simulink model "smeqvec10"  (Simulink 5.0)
settings: Solver=ode45  StartTime=0.0  StopTime=5  MaxStep=.05  RelTol=1e-4  AbsTol=1e-4
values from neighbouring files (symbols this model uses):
  Bm = 0.10    (= 0.1)    [IMabc2.m]    (also in imabcparam.m = 0.01; IMabcrun0.m = 0.01; IMabcrun1.m = 0.001; IMcur0.m = 1e-06)
  H = 0.60    (= 0.6)    [IMabc2.m]    (also in IMcur0.m = 0.3; imdef0vec.m = 0.3; imdef1vec.m = 0.3; imdef2vec.m = 0.3)
  Ra = .95    (= 0.95)    [altwdgs.m]    (also in Ccurverun.m = 0.018)
  V = [Vas 0 0].'    [Actac.m]    (also in acttrcalc1.m = str2num(get(h,'string')); im3d.m = eval(get(hVs,'String')); IMabc2.m = [vas vbs vcs 0 0 0]'; IMabcf0.m = [vas vbs vcs 0 0 0]')
  wo = 2*pi*freq0    [calc0.m]    (also in IMabc2.m = 376.991118431; imabcparam.m = 376.991118431; IMabcrun0.m = 376.991118431; IMabcrun1.m = 376.991118431)
undefined symbols (not defined in the file or in its folder): delta0, fa0, fk0, L_1, Lline, phif0, Rf, Rkd, Rkq, Rline, vs0
libraries: simulink x3

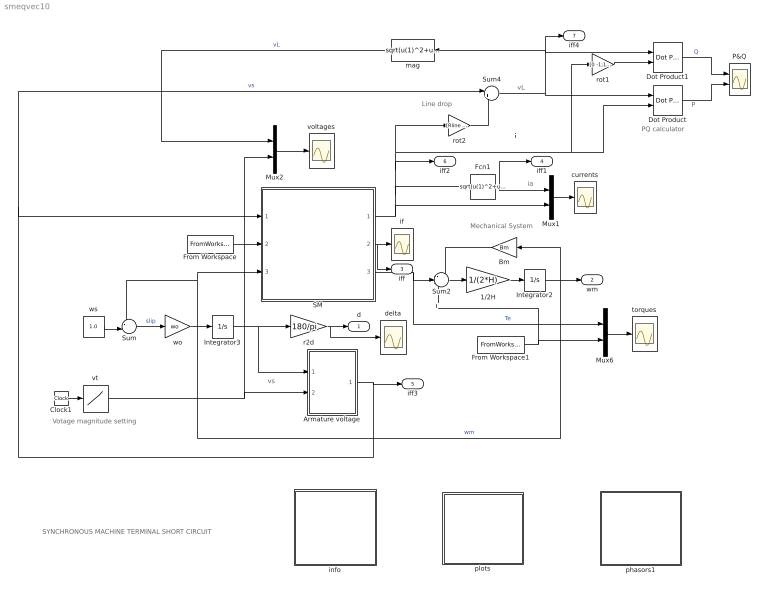
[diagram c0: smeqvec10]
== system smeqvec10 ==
  note: Tl
  note: P
  note: SYNCHRONOUS MACHINE TERMINAL SHORT CIRCUIT
  note: vs
  note: Mechanical System
  note: ia
  note: Votage magnitude setting
  note: PQ calculator
  note: vL
  note: i
  note: Line drop
  1/2H : Gain  Gain=1/(2*H)
  Armature voltage : Subsystem
  Bm : Gain  Orientation=left  Gain=Bm
  Clock1 : Clock
  Dot Product : simulink/Math Operations/Dot Product
  Dot Product1 : simulink/Math Operations/Dot Product
  Fcn1 : Fcn  Expr=sqrt(u(1)^2+u(2)^2)
  From Workspace : FromWorkspace  VariableName=vf0  SampleTime=0
  From Workspace1 : FromWorkspace  VariableName=Tl0  SampleTime=0
  Integrator2 : Integrator  InitialCondition=1
  Integrator3 : Integrator  InitialCondition=delta0
  Mux1 : Mux  Inputs=2
  Mux2 : Mux  Inputs=2
  Mux6 : Mux  Inputs=2
  P&Q : Scope  NumInputPorts=2
  SM : Subsystem
  Sum : Sum  Inputs=-+|
  Sum2 : Sum  Inputs=-+-
  Sum4 : Sum  Inputs=|++
  currents : Scope
  delta : Scope
  if : Scope
  info : Subsystem
  mag : Fcn  Orientation=left  Expr=sqrt(u(1)^2+u(2)^2)
  phasors1 : Subsystem
  plots : Subsystem
  r2d : Gain  Gain=180/pi
  rot1 : Gain  Gain=[0 -1;1 0]  Multiplication=Matrix(K*u)
  rot2 : Gain  Gain=[Rline -Lline;Lline Rline]  Multiplication=Matrix(K*u)
  torques : Scope
  voltages : Scope
  vt : Lookup  InputValues=[0 1 1.01 1.35 1.36 10 ]  OutputValues=[vs0 vs0 0 0 V V]
  wo : Gain  Gain=wo
  ws : Constant  Value=1.0
  d : Outport
  wm : Outport  Port=2
  iff : Outport  Port=3
  iff1 : Outport  Port=4
  iff3 : Outport  Port=5
  iff2 : Outport  Port=6
  iff4 : Outport  Port=7
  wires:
  1/2H/1 -> Integrator2/1
  Sum2/1 -> 1/2H/1
  Bm/1 -> Sum2/1
  SM/3(Te) -> Mux6/1, Sum2/2  "Te"
  Mux6/1 -> torques/1
  SM/1(ia) -> Mux1/2, Fcn1/1, iff2/1, rot1/1, Dot Product/2, rot2/1
  SM/2(if) -> if/1, iff/1
  Integrator2/1 -> Bm/1, wm/1, SM/3(wm), Sum/1  "wm"
  Dot Product/1 -> P&Q/2
  Dot Product1/1 -> P&Q/1  "Q"
  rot1/1 -> Dot Product1/2
  Fcn1/1 -> iff1/1, Mux1/1
  Mux1/1 -> currents/1
  r2d/1 -> delta/1, d/1
  From Workspace/1 -> SM/2(vf)
  Armature voltage/1(vs) -> iff3/1, SM/1(vs), Sum4/1  "vs"
  ws/1 -> Sum/2
  Sum/1 -> wo/1  "slip"
  wo/1 -> Integrator3/1
  Clock1/1 -> vt/1
  Sum4/1 -> Dot Product/1, Dot Product1/1, iff4/1, mag/1
  rot2/1 -> Sum4/2
  vt/1 -> Armature voltage/2(Vt), Mux2/2
  mag/1 -> Mux2/1  "vL"
  Mux2/1 -> voltages/1
  From Workspace1/1 -> Mux6/2, Sum2/3
  Integrator3/1 -> r2d/1, Armature voltage/1(delta)

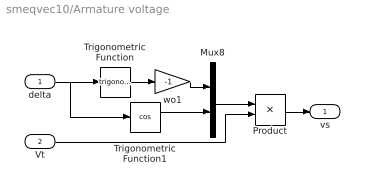
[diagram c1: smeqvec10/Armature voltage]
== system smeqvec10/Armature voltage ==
  delta : Inport
  Vt : Inport  Port=2
  Mux8 : Mux  Inputs=2
  Product : Product
  Trigonometric Function : Trigonometry
  Trigonometric Function1 : Trigonometry  Operator=cos
  wo1 : Gain  Gain=-1
  vs : Outport
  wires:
  delta/1 -> Trigonometric Function/1, Trigonometric Function1/1
  Trigonometric Function/1 -> wo1/1
  Mux8/1 -> Product/1
  wo1/1 -> Mux8/1
  Trigonometric Function1/1 -> Mux8/2
  Product/1 -> vs/1
  Vt/1 -> Product/2

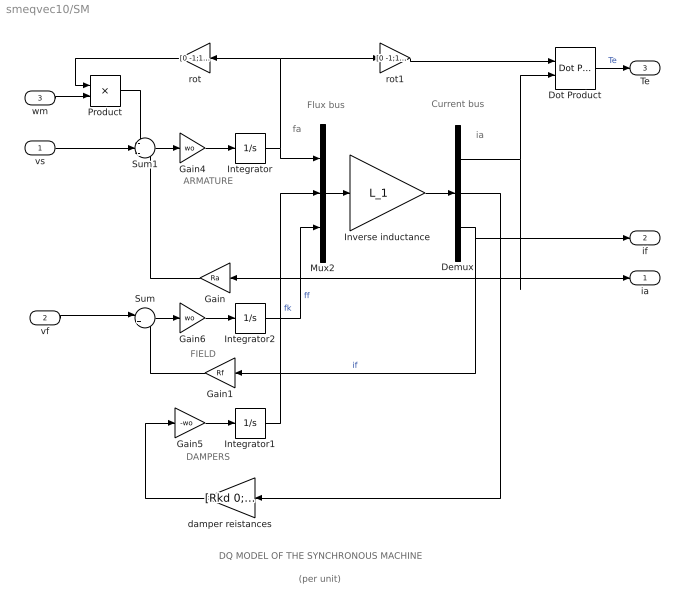
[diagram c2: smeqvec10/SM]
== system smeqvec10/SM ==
  note: DAMPERS
  note: ARMATURE
  note: fa
  note: ia
  note: FIELD
  note: DQ MODEL OF THE SYNCHRONOUS MACHINE
  note: Flux bus
  note: Current bus
  note: (per unit)
  vs : Inport
  vf : Inport  Port=2
  wm : Inport  Port=3
  Demux : Demux  Outputs=3
  Dot Product : simulink/Math Operations/Dot Product
  Gain : Gain  Orientation=left  Gain=Ra
  Gain1 : Gain  Orientation=left  Gain=Rf
  Gain4 : Gain  Gain=wo
  Gain5 : Gain  Gain=-wo
  Gain6 : Gain  Gain=wo
  Integrator : Integrator  InitialCondition=fa0
  Integrator1 : Integrator  InitialCondition=fk0
  Integrator2 : Integrator  InitialCondition=phif0
  Inverse inductance : Gain  Gain=L_1  Multiplication=Matrix(K*u)
  Mux2 : Mux  Inputs=3
  Product : Product
  Sum : Sum  Inputs=|+-
  Sum1 : Sum  Inputs=-+-
  damper reistances : Gain  Orientation=left  Gain=[Rkd 0;0 Rkq]  Multiplication=Matrix(K*u)
  rot : Gain  Orientation=left  Gain=[0 -1;1 0]  Multiplication=Matrix(K*u)
  rot1 : Gain  Gain=[0 -1;1 0]  Multiplication=Matrix(K*u)
  ia : Outport
  if : Outport  Port=2
  Te : Outport  Port=3
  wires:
  Product/1 -> Sum1/1
  rot/1 -> Product/1
  wm/1 -> Product/2
  Gain5/1 -> Integrator1/1
  damper reistances/1 -> Gain5/1
  Integrator/1 -> Mux2/1, rot/1, rot1/1
  Sum1/1 -> Gain4/1
  Gain4/1 -> Integrator/1
  vs/1 -> Sum1/2
  Gain/1 -> Sum1/3
  Gain6/1 -> Integrator2/1
  Sum/1 -> Gain6/1
  vf/1 -> Sum/1
  Gain1/1 -> Sum/2
  rot1/1 -> Dot Product/1
  Demux/1 -> Gain/1, ia/1, Dot Product/2
  Dot Product/1 -> Te/1  "Te"
  Mux2/1 -> Inverse inductance/1
  Inverse inductance/1 -> Demux/1
  Integrator1/1 -> Mux2/2  "fk"
  Integrator2/1 -> Mux2/3  "ff"
  Demux/2 -> damper reistances/1
  Demux/3 -> if/1, Gain1/1  "if"

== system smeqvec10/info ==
  note: The synchronous machine is operating at a loading condition previously established by running the model file . The machine is now experiencing a three-phase short circuit at the terminals of specified duration before being cleared. The ensuing transients are observed on several scopes.
  note: SYNCHRONOUS MACHINE
  note: SHORT CIRCUIT AT TERMINAL

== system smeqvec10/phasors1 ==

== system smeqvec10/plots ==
